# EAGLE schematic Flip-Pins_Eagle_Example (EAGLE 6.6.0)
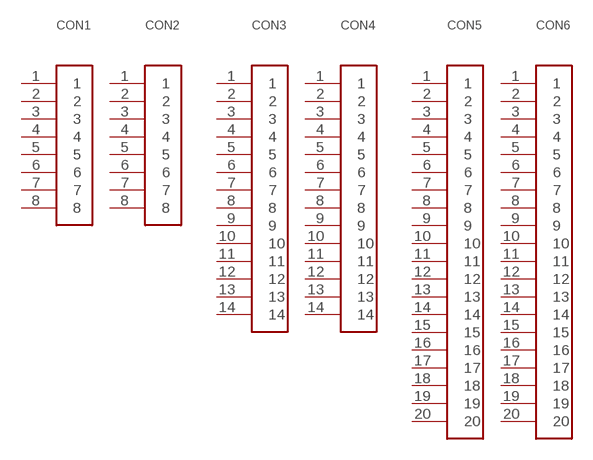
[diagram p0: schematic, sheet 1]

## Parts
CON1  FLIP-PINS-8  [FLIP-PINS-08]
CON2  FLIP-PINS-8  [FLIP-PINS-08]
CON3  FLIP-PINS-14  [FLIP-PINS-14]
CON4  FLIP-PINS-14  [FLIP-PINS-14]
CON5  FLIP-PINS-20  [FLIP-PINS-20]
CON6  FLIP-PINS-20  [FLIP-PINS-20]
Unconnected: CON1.1 CON1.2 CON1.3 CON1.4 CON1.5 CON1.6 CON1.7 CON1.8 CON2.1 CON2.2 CON2.3 CON2.4 CON2.5 CON2.6 CON2.7 CON2.8 CON3.1 CON3.2 CON3.3 CON3.4 CON3.5 CON3.6 CON3.7 CON3.8 CON3.9 CON3.10 CON3.11 CON3.12 CON3.13 CON3.14 CON4.1 CON4.2 CON4.3 CON4.4 CON4.5 CON4.6 CON4.7 CON4.8 CON4.9 CON4.10 CON4.11 CON4.12 CON4.13 CON4.14 CON5.1 CON5.2 CON5.3 CON5.4 CON5.5 CON5.6 CON5.7 CON5.8 CON5.9 CON5.10 CON5.11 CON5.12 CON5.13 CON5.14 CON5.15 CON5.16 CON5.17 CON5.18 CON5.19 CON5.20 CON6.1 CON6.2 CON6.3 CON6.4 CON6.5 CON6.6 CON6.7 CON6.8 CON6.9 CON6.10 CON6.11 CON6.12 CON6.13 CON6.14 CON6.15 CON6.16 CON6.17 CON6.18 CON6.19 CON6.20

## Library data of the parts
CON1 CON2 = Flip-Pins_Eagle_Symbols_and_Footprints_2016_09_12:FLIP-PINS-8
CON3 CON4 = Flip-Pins_Eagle_Symbols_and_Footprints_2016_09_12:FLIP-PINS-14
CON5 CON6 = Flip-Pins_Eagle_Symbols_and_Footprints_2016_09_12:FLIP-PINS-20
